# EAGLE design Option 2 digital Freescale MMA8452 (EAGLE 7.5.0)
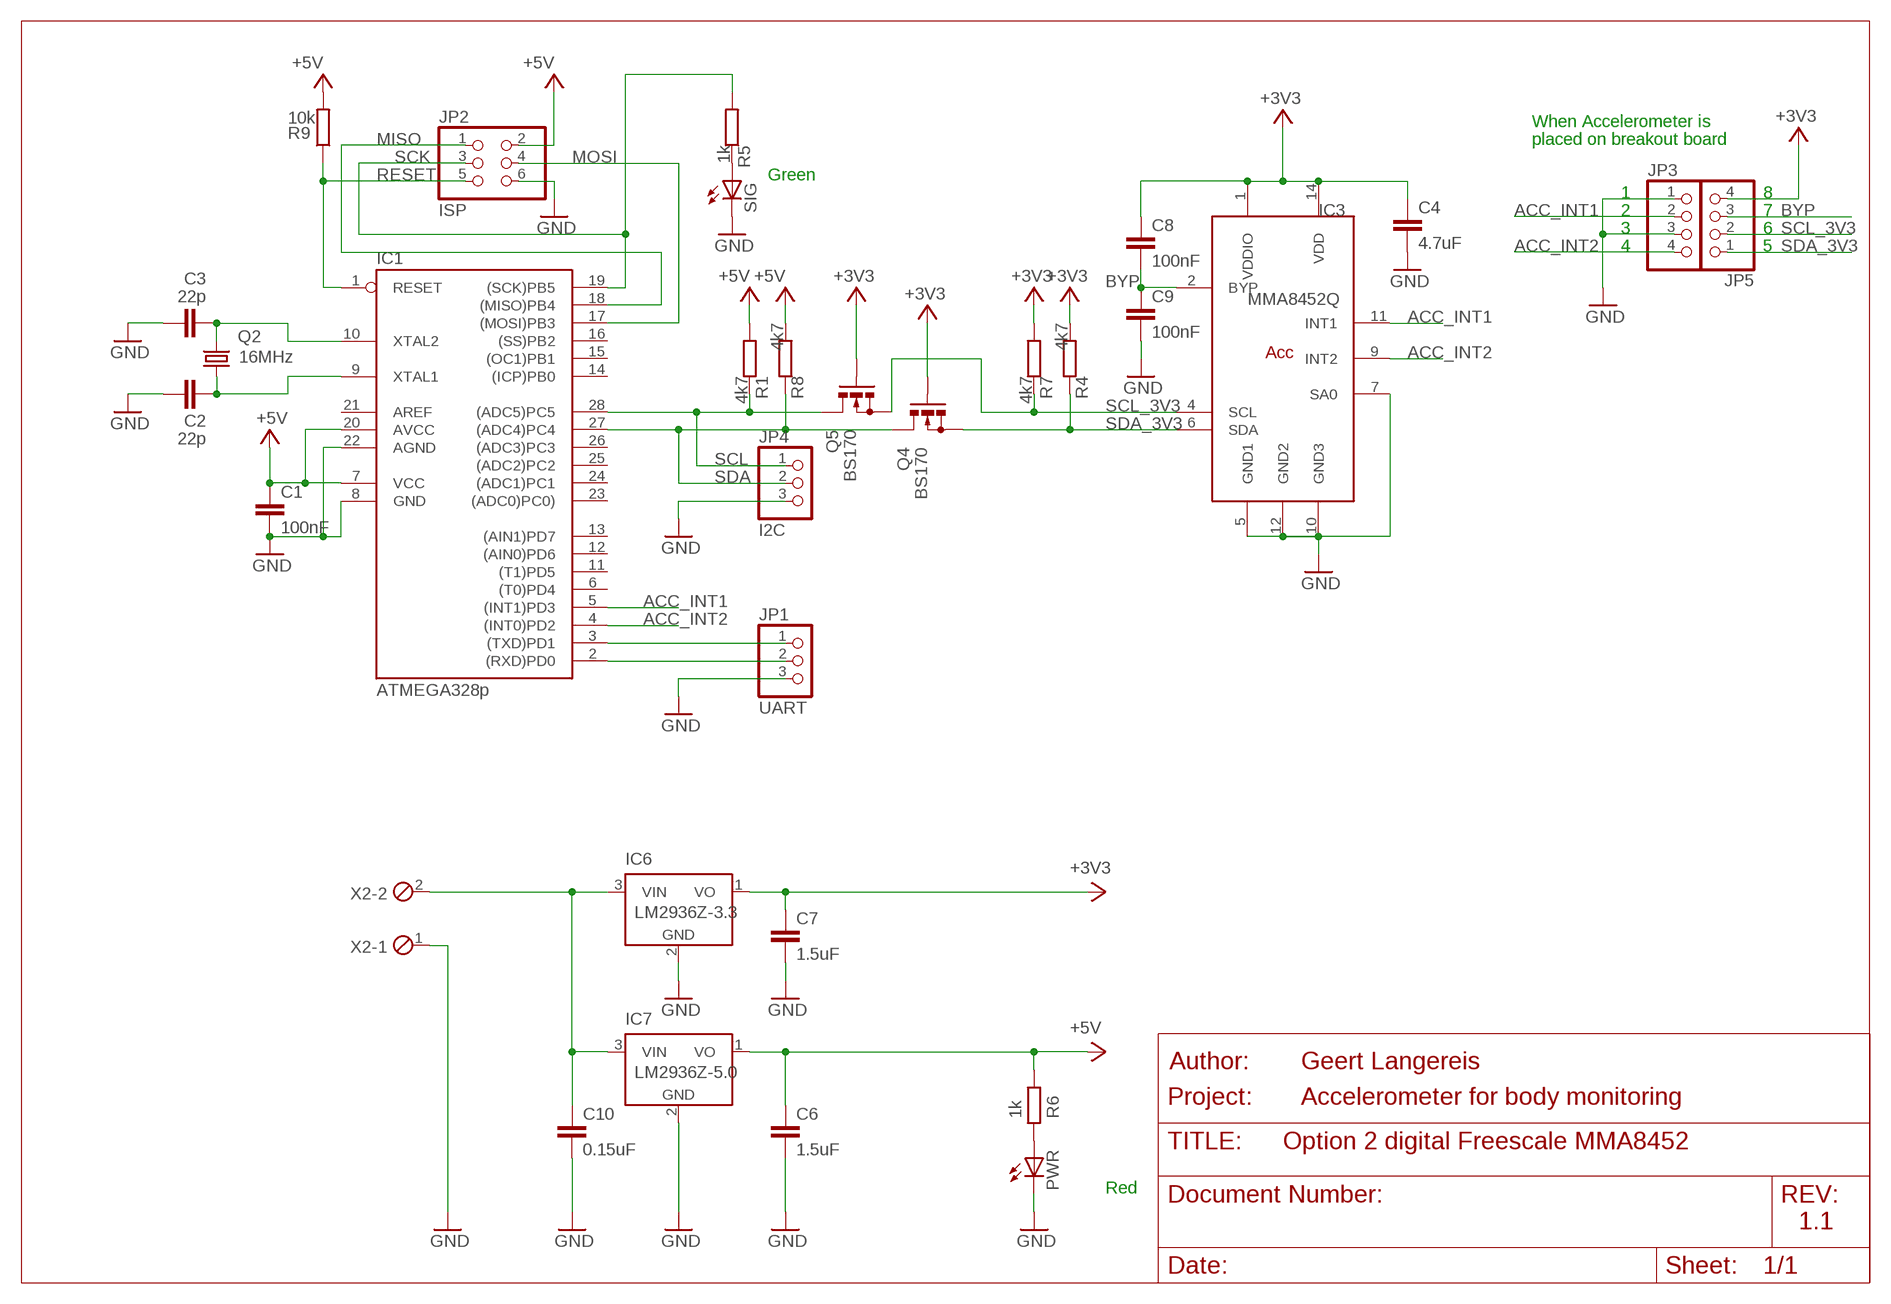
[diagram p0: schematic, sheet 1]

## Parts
C1  100nF  C5/3.5  [C5B3.5]
C2  22p  C2.5/2  [C2.5-2]
C3  22p  C2.5/2  [C2.5-2]
C4  4.7uF  C-EU050-030X075  [C050-030X075]
C6  1.5uF  C5/3.5  [C5B3.5]
C7  1.5uF  C5/3.5  [C5B3.5]
C8  100nF  C-EU050-030X075  [C050-030X075]
C9  100nF  C-EU050-030X075  [C050-030X075]
C10  0.15uF  C5/3.5  [C5B3.5]
IC1  ATMEGA328p  AT90S4433P  [DIL28-3]
IC3  MMA8452Q  [QFN-16]
IC6  LM2936Z-3.3  [TO92]
IC7  LM2936Z-5.0  [TO92]
JP1  UART  PINHD-1X3  [1X03]
JP2  ISP  PINHD-2X3  [2X03]
JP3  PINHD-1X4  [1X04]
JP4  I2C  PINHD-1X3  [1X03]
JP5  PINHD-1X4  [1X04]
PWR  LED3MM  [LED3MM]
Q2  16MHz  CRYTALHC49S  [HC49/S]
Q4  BS170  [SOT54E]
Q5  BS170  [SOT54E]
R1  4k7  R-EU_0204/7  [0204/7]
R4  4k7  R-EU_0204/7  [0204/7]
R5  1k  R-EU_0204/7  [0204/7]
R6  1k  R-EU_0204/7  [0204/7]
R7  4k7  R-EU_0204/7  [0204/7]
R8  4k7  R-EU_0204/7  [0204/7]
R9  10k  R-EU_0204/7  [0204/7]
SIG  LED3MM  [LED3MM]
X2  MPT2  [2POL254]

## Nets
+3V3 [usbvcc]: C4.1 C7.1 C8.1 IC3.1(VDDIO) IC3.14(VDD) IC6.1(VO) JP5.4 Q4.G Q5.G R4.2 R7.2
+5V: C1.1 C6.1 IC1.7(VCC) IC1.20(AVCC) IC7.1(VO) JP2.2 R1.2 R6.1 R8.2 R9.2
+9V [usbvcc]: C10.1 IC6.3(VIN) IC7.3(VIN) X2.2
ACC_INT1: IC1.5((INT1)PD3) IC3.11(INT1) JP3.2
ACC_INT2: IC1.4((INT0)PD2) IC3.9(INT2) JP3.4
BYP: C8.2 C9.1 IC3.2(BYP) JP5.3
GND [gnd]: C1.2 C2.1 C3.1 C4.2 C6.2 C7.2 C9.2 C10.2 IC1.8(GND) IC1.22(AGND) IC3.5(GND1) IC3.7(SA0) IC3.10(GND3) IC3.12(GND2) IC6.2(GND) IC7.2(GND) JP1.3 JP2.6 JP3.1 JP3.3 JP4.3 PWR.K(C) SIG.K(C) X2.1
MISO: IC1.18((MISO)PB4) JP2.1
MOSI: IC1.17((MOSI)PB3) JP2.4
N$1: IC1.3((TXD)PD1) JP1.1
N$2: IC1.2((RXD)PD0) JP1.2
N$3: PWR.A R6.2
N$4: R5.1 SIG.A
N$6: C2.2 IC1.9(XTAL1) Q2.1
N$7: C3.2 IC1.10(XTAL2) Q2.2
RESET [usbvcc]: IC1.1(RESET) JP2.5 R9.1
SCK: IC1.19((SCK)PB5) JP2.3 R5.2
SCL: IC1.28((ADC5)PC5) JP4.1 Q5.D R1.1
SCL_3V3: IC3.4(SCL) JP5.2 Q5.S R7.1
SDA: IC1.27((ADC4)PC4) JP4.2 Q4.D R8.1
SDA_3V3: IC3.6(SDA) JP5.1 Q4.S R4.1
Unconnected: IC1.6((T0)PD4) IC1.11((T1)PD5) IC1.12((AIN0)PD6) IC1.13((AIN1)PD7) IC1.14((ICP)PB0) IC1.15((OC1)PB1) IC1.16((SS)PB2) IC1.21(AREF) IC1.23((ADC0)PC0)) IC1.24((ADC1)PC1) IC1.25((ADC2)PC2) IC1.26((ADC3)PC3)

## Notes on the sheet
- When Accelerometer is
- placed on breakout board
- Green
- 1 | 8
- 2 | 7
- 3 | 6
- 4 | 5
- Geert Langereis
- Accelerometer for body monitoring
- Red
- 1.1

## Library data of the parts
C1-C3 C6 C7 C10 = capacitor-wima:C: CAPACITOR
C4 C8 C9 = resistor:C-EU: CAPACITOR, European symbol
IC1 = atmel:AT90S4433: MICROCONTROLLER 4 Kbytes FLASH 128 bytes SRAM 256 bytes EEPROM UART 6-channel 10 bit ADC; OC_FARNELL: unknown; OC_NEWARK: unknown
IC3 = Geert-library:MMA8452Q: 3-Axis, 12-bit/8-bit Digital Accelerometer (Freescale)
IC6 = national-semiconductor:LM2936?*: Ultra-Low Quiescent Current LDO Voltage Regulator Source: Data sheet; MF: NATIONAL SEMICONDUCTOR; MPN: LM2936Z-3.3/NOPB; OC_FARNELL: 1564641; OC_NEWARK: 41K4532
IC7 = national-semiconductor:LM2936?*: Ultra-Low Quiescent Current LDO Voltage Regulator Source: Data sheet; MF: NATIONAL SEMICONDUCTOR; MPN: LM2936Z-5.0/NOPB; OC_FARNELL: 1150143; OC_NEWARK: 41K4533
JP1 JP4 = pinhead:PINHD-1X3: PIN HEADER
JP2 = pinhead:PINHD-2X3: PIN HEADER
JP3 JP5 = pinhead:PINHD-1X4: PIN HEADER
PWR SIG = led:LED: LED
Q2 = crystal:CRYTAL: CRYSTAL
Q4 Q5 = transistor-small-signal:BS170: N-CHANNEL MOS FET
R1 R4-R9 = resistor:R-EU_: RESISTOR, European symbol
X2 = con-phoenix-254:MPT2: PHOENIX CONNECTOR; OC_FARNELL: unknown; OC_NEWARK: unknown

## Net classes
0 default: width 0.254 mm, drill 0.305 mm, clearance 0.152 mm
1 power: width 0.61 mm, drill 0.508 mm, clearance 0.152 mm
2 gnd: width 0.305 mm, drill 0.508 mm, clearance 0.152 mm
3 usbvcc: width 0.508 mm, drill 0.508 mm, clearance 0.152 mm
4 aref: width 0.406 mm

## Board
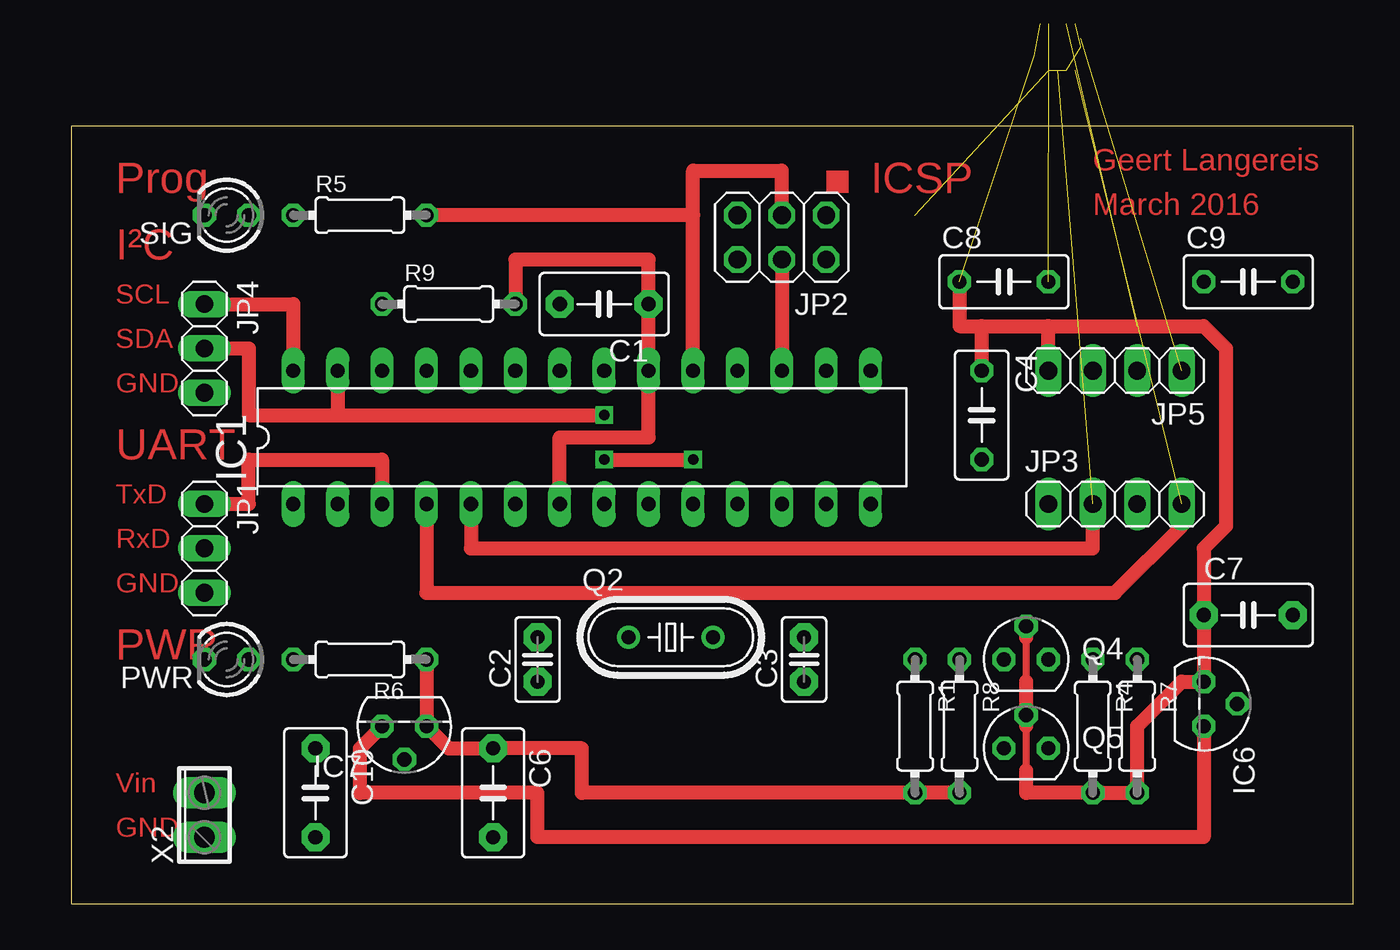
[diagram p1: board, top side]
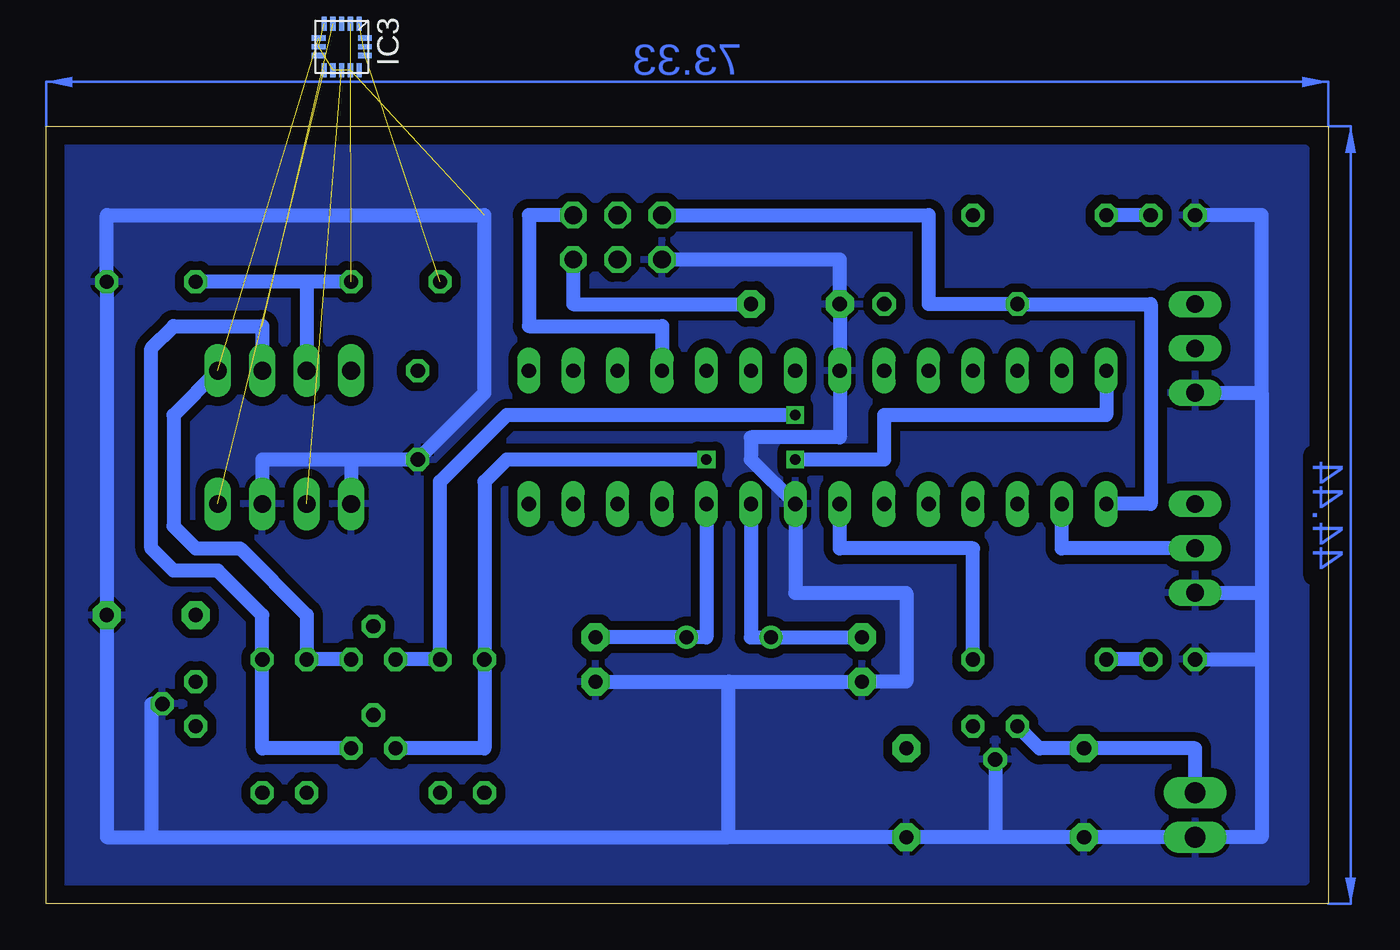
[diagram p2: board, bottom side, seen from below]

Size 73.33 x 44.44 mm. Coordinates in mm from the lower left corner, seen from the top.
Outline: 0,0 73.33,0 73.33,44.44 0,44.44 0,0
Copper layers (1*16): Top 0.035mm / dielectric 1.5mm / Bottom 0.035mm
Design rules "default *": minimum track width 10mil, minimum drill 24mil, track to track 20mil, track to pad 20mil, pad to pad 20mil, via to via 20mil, smd to smd 8mil, copper to edge 40mil, drill to drill 8mil, minimum pad ring 10mil, minimum via ring 8mil, stop-mask expansion 4mil, vias tented up to drill 0mil, thermal gap 10mil

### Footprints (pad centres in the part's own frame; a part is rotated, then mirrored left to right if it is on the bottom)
C5B3.5 = drill 0.813 pad 1.6 octagon: 1 -2.54,0; 2 2.54,0
C2.5-2 = drill 0.813 pad 1.6 octagon: 1 -1.27,0; 2 1.27,0
C050-030X075 = drill 0.813 octagon: 1 -2.54,0; 2 2.54,0
DIL28-3 = drill 0.813 long: 1 -16.51,-3.81; 2 -13.97,-3.81; 3 -11.43,-3.81; 4 -8.89,-3.81; 5 -6.35,-3.81; 6 -3.81,-3.81; 7 -1.27,-3.81; 8 1.27,-3.81; 9 3.81,-3.81; 10 6.35,-3.81; 11 8.89,-3.81; 12 11.43,-3.81; 13 13.97,-3.81; 14 16.51,-3.81; 15 16.51,3.81; 16 13.97,3.81; 17 11.43,3.81; 18 8.89,3.81; 19 6.35,3.81; 20 3.81,3.81; 21 1.27,3.81; 22 -1.27,3.81; 23 -3.81,3.81; 24 -6.35,3.81; 25 -8.89,3.81; 26 -11.43,3.81; 27 -13.97,3.81; 28 -16.51,3.81
QFN-16 = smd 0.8 x 0.3: 1 -3.325,3; 2 -3.325,2.5; 3 -3.325,2; 4 -3.325,1.5; 5 -3.325,1; 9 -0.675,1; 10 -0.675,1.5; 11 -0.675,2; 12 -0.675,2.5; 13 -0.675,3 | smd 0.3 x 0.8: 6 -2.5,0.675; 7 -2,0.675; 8 -1.5,0.675; 14 -1.5,3.325; 15 -2,3.325; 16 -2.5,3.325
TO92 = drill 0.813 pad 1.27 octagon: 1 -1.27,0; 2 0,1.905; 3 1.27,0
1X03 = drill 1.016 long: 1 -2.54,0; 2 0,0; 3 2.54,0
2X03 = drill 1.016 octagon: 1 -2.54,-1.27; 2 -2.54,1.27; 3 0,-1.27; 4 0,1.27; 5 2.54,-1.27; 6 2.54,1.27
1X04 = drill 1.016 long: 1 -3.81,0; 2 -1.27,0; 3 1.27,0; 4 3.81,0
LED3MM = drill 0.813 octagon: A -1.27,0; K 1.27,0
HC49/S = drill 0.813: 1 -2.413,0; 2 2.413,0
SOT54E = drill 0.813 octagon: D -1.27,0; G 0,1.905; S 1.27,0
0204/7 = drill 0.813 octagon: 1 -3.81,0; 2 3.81,0
2POL254 = drill 1.2 long: 1 -1.27,0; 2 1.27,0

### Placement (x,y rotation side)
C1  30.48,34.29 180 top
C2  26.67,13.97 90 top
C3  41.91,13.97 90 top
C4  52.07,27.94 270 top
C6  24.13,6.35 270 top
C7  67.31,16.51 0 top
C8  53.34,35.56 0 top
C9  67.31,35.56 0 top
C10  13.97,6.35 270 top
IC1  29.21,26.67 0 top
IC3  not placed on the board
IC6  64.77,11.43 270 top
IC7  19.05,10.16 180 top
JP1  7.62,20.32 270 top
JP2  40.64,38.1 180 top
JP3  59.69,22.86 0 top
JP4  7.62,31.75 270 top
JP5  59.69,30.48 180 top
PWR  8.89,13.97 180 top
Q2  34.29,15.24 0 top
Q4  54.61,13.97 0 top
Q5  54.61,8.89 0 top
R1  48.26,10.16 270 top
R4  58.42,10.16 270 top
R5  16.51,39.37 0 top
R6  16.51,13.97 180 top
R7  60.96,10.16 270 top
R8  50.8,10.16 270 top
R9  21.59,34.29 0 top
SIG  8.89,39.37 180 top
X2  7.62,5.08 90 top

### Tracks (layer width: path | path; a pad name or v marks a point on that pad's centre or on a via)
+3V3  (2 unrouted)
  Top 0.406: 54.61,7.62 54.61,10.16 | 54.61,12.7 54.61,15.24
  Top 0.813: 54.61,7.62 54.61,6.35 R4.2 R7.2 60.96,10.16 63.5,12.7 IC6.1 C7.1 64.77,20.32 66.04,21.59 66.04,31.75 64.77,33.02 55.88,33.02 | 54.61,10.16 Q5.G 54.61,12.7 | 54.61,15.24 Q4.G | JP5.4 55.88,33.02 | C8.1 50.8,33.02 52.07,33.02 | 52.07,33.02 55.88,33.02 | C4.1 52.07,33.02
+5V
  Top 0.813: R6.1 IC7.1 21.59,8.89 C6.1 29.21,8.89 29.21,6.35 R1.2 R8.2 | IC1.7 27.94,26.67 33.02,26.67 IC1.20 C1.1 33.02,36.83 25.4,36.83 R9.2
  Bottom 0.813: R6.1 20.32,20.32 27.94,20.32 IC1.7 | JP2.2 43.18,34.29 C1.1
+9V
  Top 0.813: IC6.3 64.77,3.81 26.67,3.81 26.67,6.35 16.51,6.35 16.51,8.89 IC7.3
  Bottom 0.813: X2.2 7.62,8.89 C10.1 16.51,8.89 IC7.3
ACC_INT1  (1 unrouted)
  Top 0.813: IC1.5 22.86,20.32 58.42,20.32 JP3.2
ACC_INT2  (1 unrouted)
  Top 0.813: IC1.4 20.32,17.78 59.69,17.78 63.5,21.59 JP3.4
BYP  (1 unrouted)
  Bottom 0.813: C9.1 C8.2 58.42,35.56 JP5.3
GND  (4 unrouted)
  Bottom 0.813: 19.05,3.81 C10.2 X2.1 3.81,3.81 3.81,13.97 | 19.05,3.81 C6.2 34.29,3.81 | JP2.6 27.94,36.83 C1.2 IC1.22 27.94,26.67 33.02,26.67 33.02,25.4 IC1.8 30.48,17.78 24.13,17.78 24.13,12.7 C2.1 34.29,12.7 | C3.1 34.29,12.7 | 67.31,3.81 69.85,3.81 C7.2 C9.2 69.85,39.37 48.26,39.37 48.26,29.21 C4.2 55.88,25.4 | 67.31,3.81 34.29,3.81 | IC6.2 67.31,11.43 67.31,3.81 | IC7.2 19.05,3.81 | 34.29,3.81 34.29,12.7 | 3.81,29.21 3.81,17.78 | 3.81,17.78 3.81,13.97 | JP4.3 3.81,29.21 | 3.81,29.21 3.81,39.37 SIG.K | PWR.K 3.81,13.97 | JP1.3 3.81,17.78 | 55.88,25.4 JP3.1 | 55.88,25.4 60.96,25.4 JP3.3
  pour Bottom: 1.27,43.18 72.39,43.18 72.39,1.27 1.27,1.27
MISO
  Bottom 0.813: JP2.1 45.72,39.37 45.72,33.02 38.1,33.02 IC1.18
MOSI
  Top 0.813: JP2.4 IC1.17
N$1
  Top 0.813: JP1.1 10.16,22.86 10.16,25.4 17.78,25.4 IC1.3
N$2
  Bottom 0.813: JP1.2 15.24,20.32 IC1.2
N$3
  Bottom 0.813: PWR.A R6.2
N$4
  Bottom 0.813: SIG.A R5.1
N$6
  Bottom 0.813: IC1.9 33.02,15.24 Q2.1 C2.2
N$7
  Bottom 0.813: IC1.10 35.56,15.24 Q2.2 C3.2
RESET
  Bottom 0.813: JP2.5 22.86,39.37 22.86,34.29 R9.1 10.16,34.29 10.16,22.86 IC1.1
SCK
  Top 0.813: 35.56,39.37 35.56,41.91 40.64,41.91 JP2.3 | IC1.19 35.56,39.37 | 35.56,39.37 R5.2
SCL  (via drill 0.6)
  Top 0.813: JP4.1 12.7,34.29 IC1.28 | v30.48,25.4 v35.56,25.4
  Bottom 0.813: Q5.D 48.26,8.89 R1.1 48.26,24.13 46.99,25.4 v35.56,25.4 | IC1.28 12.7,27.94 25.4,27.94 25.4,25.4 v30.48,25.4
SCL_3V3  (1 unrouted)
  Bottom 0.813: Q5.S 60.96,8.89 R7.1 60.96,16.51 63.5,19.05 66.04,19.05 67.31,20.32 67.31,31.75 66.04,33.02 60.96,33.02 JP5.2
SDA  (via drill 0.6)
  Top 0.813: JP4.2 10.16,31.75 10.16,27.94 15.24,27.94 | IC1.27 15.24,27.94 | 15.24,27.94 v30.48,27.94
  Bottom 0.813: Q4.D R8.1 50.8,24.13 46.99,27.94 v30.48,27.94
SDA_3V3  (1 unrouted)
  Bottom 0.813: Q4.S R4.1 58.42,16.51 62.23,20.32 64.77,20.32 66.04,21.59 66.04,27.94 JP5.1
(copper drawn outside any net)
  shapes: Bottom area x2, Top area x1

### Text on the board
Top: Geert Langereis | Prog | ICSP | March 2016 | I²C | SCL | SDA | GND | UART | TxD | RxD | GND | PWR | Vin | GND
